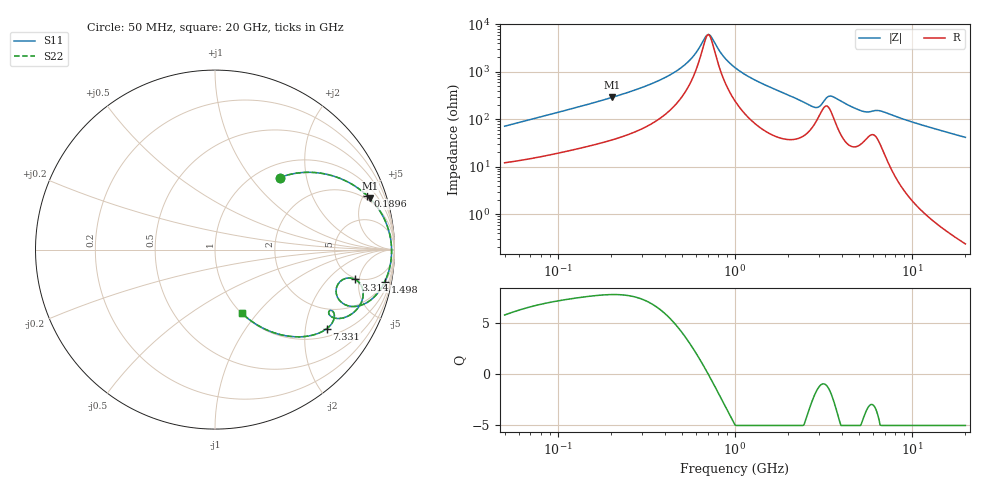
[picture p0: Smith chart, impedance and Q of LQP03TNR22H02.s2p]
!Murata Part Number: LQP03TNR22H02
!These Parameters are Measured in Series Mode Connection
!  o--[Z]--o
!Port1  Port2
!  o-------o
!Freq. Start=50[MHz] Stop=20[GHz], 401[Steps]
# Hz S RI R 50
!Freq.(Hz) S11(Real) S11(Imag) S21(Real) S21(Imag) S12(Real) S12(Imag) S22(Real) S22(Imag)
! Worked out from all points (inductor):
!   401 points, 50 MHz to 20 GHz, reference 50 ohm
!   read as one part in series: L = 221 nH near 51.52 MHz
!   highest Q = 7.8 at 201.3 MHz (marker M1), where L = 225 nH
!   self-resonance near 698 MHz
!   S11 on the Smith chart (normalised r, x): 50 MHz: 1.24, +1.41; 189.6 MHz: 1.69, +5.34; 1.498 GHz: 2, -10; 3.314 GHz: 4.79, -4.40; 7.331 GHz: 1.24, -2.62; 20 GHz: 1.00, -0.83
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5e7  0.3602 0.4015  0.6398 -0.4015  0.6398 -0.4015  0.3602 0.4015
1.364002e8  0.7559 0.3683  0.2441 -0.3683  0.2441 -0.3683  0.7559 0.3683
1.896393e8  0.8495 0.2991  0.1505 -0.2991  0.1505 -0.2991  0.8495 0.2991
2.013488e8  0.8634 0.2853  0.1366 -0.2853  0.1366 -0.2853  0.8634 0.2853
3.721004e8  0.9563 0.1409  0.0437 -0.1409  0.0437 -0.1409  0.9563 0.1409
5.330693e8  0.9783 0.0609  0.0217 -0.0609  0.0217 -0.0609  0.9783 0.0609
7.08568e8  0.9839 -0.000527  0.0161 0.000527  0.0161 0.000527  0.9839 -0.000527
8.608917e8  0.9824 -0.0432  0.0176 0.0432  0.0176 0.0432  0.9824 -0.0432
1e9  0.978 -0.0771  0.022 0.0771  0.022 0.0771  0.978 -0.0771
1.498439e9  0.9461 -0.1786  0.0539 0.1786  0.0539 0.1786  0.9461 -0.1786
2.146657e9  0.8633 -0.284  0.1367 0.284  0.1367 0.284  0.8633 -0.284
2.728004e9  0.7121 -0.2997  0.2879 0.2997  0.2879 0.2997  0.7121 -0.2997
2.98453e9  0.6772 -0.211  0.3228 0.211  0.3228 0.211  0.6772 -0.211
3.314454e9  0.7812 -0.1666  0.2188 0.1666  0.2188 0.1666  0.7812 -0.1666
3.736399e9  0.8245 -0.263  0.1755 0.263  0.1755 0.263  0.8245 -0.263
4.472136e9  0.7523 -0.3645  0.2477 0.3645  0.2477 0.3645  0.7523 -0.3645
5.433528e9  0.6401 -0.3666  0.3599 0.3666  0.3599 0.3666  0.6401 -0.3666
6.034176e9  0.6489 -0.3392  0.3511 0.3392  0.3511 0.3392  0.6489 -0.3392
7.331367e9  0.6226 -0.4406  0.3774 0.4406  0.3774 0.4406  0.6226 -0.4406
7.442007e9  0.6142 -0.4467  0.3858 0.4467  0.3858 0.4467  0.6142 -0.4467
1.082228e10  0.3924 -0.4796  0.6076 0.4796  0.6076 0.4796  0.3924 -0.4796
2e10  0.1488 -0.3531  0.8512 0.3531  0.8512 0.3531  0.1488 -0.3531
